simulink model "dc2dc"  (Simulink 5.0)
settings: Solver=ode45  StartTime=0.0  StopTime=5e-5  MaxStep=1e-7  RelTol=1e-3
libraries: simulink x1

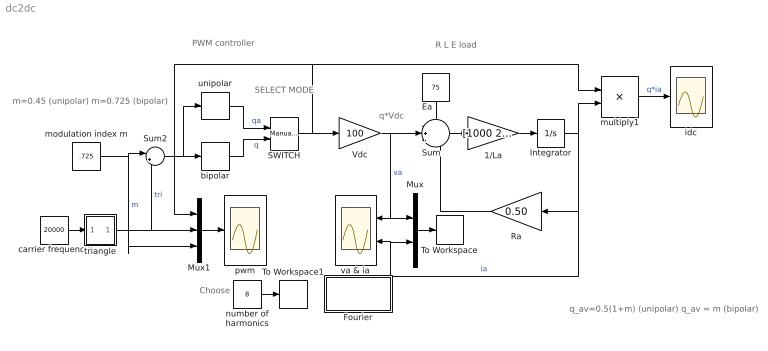
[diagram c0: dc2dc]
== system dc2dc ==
  note: PWM controller
  note: Choose
  note: R L E load
  note: q*Vdc
  note: m=0.45 (unipolar) m=0.725 (bipolar)
  note: q_av=0.5(1+m) (unipolar) q_av = m (bipolar)
  note: SELECT MODE
  1/La : Gain  Gain=[1000 200]
  Ea : Constant  Orientation=down  Value=75
  Fourier : Subsystem
  Integrator : Integrator  InitialCondition=-5.0
  Mux : Mux  Inputs=2
  Mux1 : Mux  Inputs=3
  Ra : Gain  Orientation=left  Gain=0.50
  SWITCH : simulink/Signal Routing/Manual Switch  sw=0  action=0
  Sum : Sum  Inputs=-+-
  Sum2 : Sum  Inputs=|+-
  To Workspace : ToWorkspace  VariableName=f  SampleTime=-1  SaveFormat=Array
  To Workspace1 : ToWorkspace  VariableName=h  SampleTime=-1  SaveFormat=Array
  Vdc : Gain  Gain=100
  bipolar : Signum
  carrier frequency : Constant  Value=20000
  idc : Scope
  modulation index m : Constant  Value=.725
  multiply1 : Product
  number of harmonics : Constant  Value=8
  pwm : Scope
  triangle : Subsystem
  unipolar : Relay
  va & ia : Scope  NumInputPorts=2
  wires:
  Ra/1 -> Sum/3
  Sum/1 -> 1/La/1
  1/La/1 -> Integrator/1
  Ea/1 -> Sum/1
  Vdc/1 -> Sum/2, Mux/1, va & ia/1  "va"
  modulation index m/1 -> Sum2/1, Mux1/3  "m"
  Integrator/1 -> multiply1/2, Ra/1, Mux/2, va & ia/2  "ia"
  multiply1/1 -> idc/1  "q*ia"
  Mux/1 -> To Workspace/1
  Mux1/1 -> pwm/1
  carrier frequency/1 -> triangle/1(fc)
  triangle/1(tri) -> Mux1/2, Sum2/2  "tri"
  Sum2/1 -> bipolar/1, unipolar/1
  number of harmonics/1 -> To Workspace1/1
  SWITCH/1 -> Vdc/1, multiply1/1, Mux1/1
  bipolar/1 -> SWITCH/2  "q"
  unipolar/1 -> SWITCH/1  "qa"

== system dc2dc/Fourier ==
  note: To obtain the Fourier decomposition of a periodic signal: a) run a simulation for one period duration b) Specify the fundamental frequency c) Specify the number of harmonics

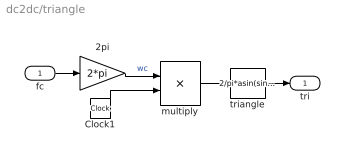
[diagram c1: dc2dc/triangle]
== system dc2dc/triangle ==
  fc : Inport
  2pi : Gain  Gain=2*pi
  Clock1 : Clock
  multiply : Product
  triangle : Fcn  Expr=2/pi*asin(sin(u-pi/2))
  tri : Outport
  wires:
  Clock1/1 -> multiply/2
  multiply/1 -> triangle/1
  fc/1 -> 2pi/1
  triangle/1 -> tri/1
  2pi/1 -> multiply/1  "wc"
